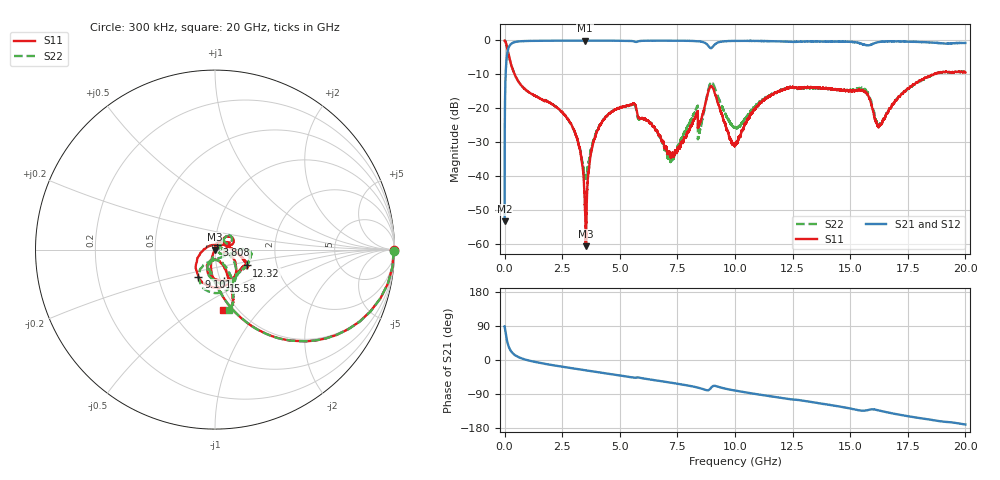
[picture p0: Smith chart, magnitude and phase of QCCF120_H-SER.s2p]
!{QCCF120}
!Johanson Technology Inc.
!www.johansontechnology.com
!Test Board Conditions:
!Substrate Type  RO4350B
!Substrate Thickness  10 mil
!Substrate Dk  3.66
!TL Type: GCPW
!TL Trace Width  21 mil
!TL Gap  20 mil
!Electrode orientation  Horizontal
!DUT TOPOLOGY	SERIES
!Mounting Pad LxW  16x21 mil
! Created Sat Jan  9 18:18:28 2021
# hz S ma R 50
! 2 Port Network Data from SP1.SP block
! freq  magS11  angS11  magS21  angS21  magS12  angS12  magS22  angS22
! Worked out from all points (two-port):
!   20001 points, 300 kHz to 20 GHz, reference 50 ohm
!   highest |S21| = -0.03 dB at 3.488 GHz (marker M1); lowest = -53.2 dB at 300 kHz (marker M2)
!   |S21| within 3 dB of the highest: 137.4 MHz to end of sweep
!   lowest |S11| = -60.5 dB at 3.529 GHz (marker M3), VSWR 1.00, Z = 49.9 + j0.0462 ohm
!   |S11| at or under -10 dB: 436.8 MHz to 18.62 GHz (18.18 GHz wide, 191 % of centre)
!   |S22| runs from -40.7 to 0.0 dB; largest |S21 - S12| = 0.012
!   S11 on the Smith chart (normalised r, x): 300 kHz: open; 3.808 GHz: 1.02, +0.05; 9.101 GHz: 0.80, -0.25; 12.32 GHz: 1.40, -0.26; 15.58 GHz: 1.04, -0.37; 20 GHz: 0.86, -0.65
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300000  0.9956 -0.3  0.002185 89.3  0.002184 88.9  0.9966 -0.4
1.073e8  0.7837 -39.4  0.6166 50.4  0.6176 50.3  0.7846 -39.4
2.513e8  0.4818 -63.6  0.8708 25.9  0.8722 25.9  0.4831 -63.6
2.7033e9  0.0723 -106.8  0.9943 -19.6  0.9956 -19.6  0.07218 -108.7
3.3343e9  0.0182 -116.6  0.9958 -25.5  0.996 -25.5  0.01913 -90.2
3.4883e9  0.00347 -141.9  0.9968 -26.9  0.9953 -26.9  0.009492 -42.5
3.5293e9  0.0009412 150.6  0.9957 -27.3  0.9958 -27.3  0.009357 -21.5
3.8083e9  0.02733 62.9  0.9954 -29.9  0.9952 -29.9  0.02938 40.2
4.4463e9  0.07723 53.6  0.9919 -35.7  0.9933 -35.8  0.07815 49.8
5.5363e9  0.115 36.7  0.9789 -46.1  0.9794 -46.1  0.114 43.2
6.6673e9  0.04199 33.9  0.9923 -54.8  0.9928 -54.7  0.04183 45.8
7.2713e9  0.02218 72.5  0.9913 -60.4  0.9914 -60.4  0.01978 -11.9
8.2863e9  0.0762 33.0  0.9783 -71.4  0.9772 -71.3  0.09304 -16.5
8.4873e9  0.06277 -17.6  0.9677 -74.4  0.966 -74.4  0.04925 -2.2
9.1013e9  0.1766 -121.4  0.8578 -68.0  0.8565 -68.0  0.21 -111.9
1.00003e10  0.02814 91.6  0.9847 -80.7  0.9849 -80.7  0.05292 -77.1
1.23233e10  0.198 -26.5  0.9602 -102.7  0.9617 -103.0  0.1992 -4.5
1.33343e10  0.2028 -27.0  0.9639 -111.0  0.9657 -111.2  0.201 -15.4
1.55823e10  0.1797 -74.1  0.8777 -133.7  0.8754 -134.1  0.1953 -75.5
1.62033e10  0.05479 -95.9  0.9408 -132.6  0.9425 -132.5  0.05815 -94.3
1.66673e10  0.09304 -63.1  0.972 -139.0  0.9626 -138.9  0.0928 -60.8
2e10  0.3396 -83.0  0.918 -170.2  0.9106 -170.2  0.3449 -77.2
